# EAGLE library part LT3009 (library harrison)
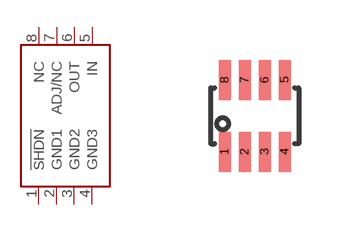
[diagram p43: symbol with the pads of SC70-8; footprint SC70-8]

Designator prefix U

## LT3009  [SC70-8]
1  !SHDN!  in
2  GND1  pwr
3  GND2  pwr
4  GND3  pwr
5  IN  pwr
6  OUT  pwr
7  ADJ/NC  pas
8  NC  nc

## Footprint SC70-8 (pad centres in mm)
smd 0.3 x 1: 1 -0.75,-0.9; 2 -0.25,-0.9; 3 0.25,-0.9; 4 0.75,-0.9; 5 0.75,0.9; 6 0.25,0.9; 7 -0.25,0.9; 8 -0.75,0.9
